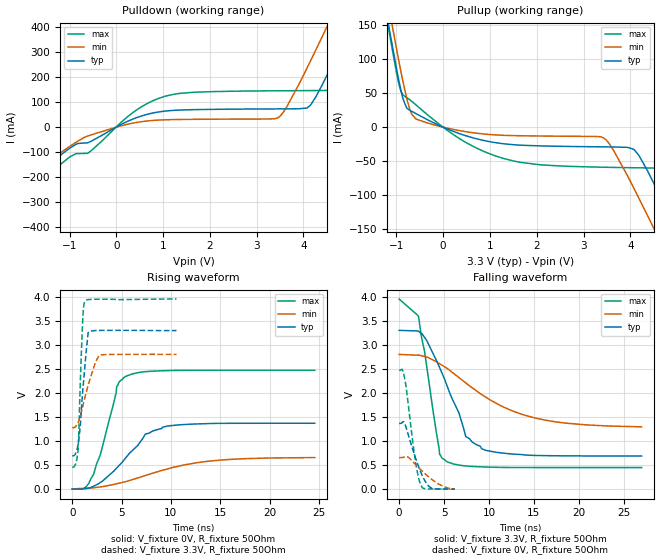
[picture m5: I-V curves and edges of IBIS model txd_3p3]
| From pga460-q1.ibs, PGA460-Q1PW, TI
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|   txd_3p3 Model
[Model]   txd_3p3
Model_type   Output
Polarity   Non-Inverting
Vmeas = 1.65
Vref = 0
Cref = 2pF
Rref = 600
|   typ   min   max
|   (nom PVT)   (fast PVT)   (slow PVT)
C_comp   1.546e-12   1.546e-12   1.546e-12
| Where nom  PVT is Nominal Process, 3.3V, 27C
|   Fast PVT is Strong Process,  3.95V, -40C
|   Slow PVT is Weak Process,   2.8V, 125C
[Voltage Range]   3.3   2.8   3.95
|Junction Temperature
[Temperature Range]   27   125   -40
[Pullup Reference]   3.3   2.8   3.95
[Pulldown Reference]   0   0   0
[Power Clamp Reference]   3.3   2.8   3.95
[GND Clamp Reference]   0   0   0
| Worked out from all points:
|   slope of the pulldown table from 0 to 0.495 V, typ, clamps not added: 11.9 ohm
|   slope of the pullup table from 0 to 0.495 V, typ, clamps not added: 38.7 ohm
|   falling waveform, V_fixture 3.3V, R_fixture 50Ohm: 20-80 % time 3.37ns typ, 7.63ns min, 1.76ns max; typ from 3.3 V to 0.689 V
|   rising waveform, V_fixture 0V, R_fixture 50Ohm: 20-80 % time 3.6ns typ, 7.01ns min, 1.99ns max; typ from 0 V to 1.37 V
|   rising waveform, V_fixture 3.3V, R_fixture 50Ohm: 20-80 % time 611ps typ, 1.23ns min, 346ps max; typ from 0.689 V to 3.29 V
|   falling waveform, V_fixture 0V, R_fixture 50Ohm: 20-80 % time 1.52ns typ, 2.39ns min, 1.01ns max; typ from 1.37 V to 0 V
[Pulldown]
|   Voltage   I(typ)   I(min)   I(max)
-3.3V     -421.7mA   -396.6mA   -469.6mA
-716.7mV  -63.75mA   -44.17mA   -104.9mA
804.8mV   57.27mA    27.04mA    107.1mA
1.647V    69.71mA    31.12mA    138.9mA
3.445V    72.68mA    36.55mA    145mA
3.633V    72.81mA    77.77mA    145.2mA
4.075V    76.37mA    235.5mA    145.7mA
4.557V    227.4mA    422.1mA    146.8mA
4.833V    334.7mA    530.8mA    152.6mA
5.046V    419.1mA    614.8mA    215mA
5.514V    608.1mA    800.5mA    399.1mA
6.6V      1.053A     1.233A     854.8mA
[Pullup]
|   Voltage   I(typ)   I(min)   I(max)
-3.3V     1.024A     1.027A     1.051A
-1.144V   141.3mA    170mA      136.2mA
-902.3mV  54.03mA    81.66mA    52.9mA
-715.6mV  24.87mA    26.75mA    40.4mA
-575.6mV  19.68mA    11.74mA    32.37mA
1.092V    -22.58mA   -11.34mA   -41.74mA
3.42V     -29.04mA   -15.47mA   -59.01mA
4.075V    -32.79mA   -89.97mA   -59.78mA
4.495V    -81.79mA   -148.1mA   -60.25mA
5.054V    -162.5mA   -227.5mA   -93.94mA
5.406V    -215mA     -277.9mA   -146.3mA
6.6V      -395.5mA   -449.7mA   -336.5mA
[Ramp]
R_load = 50
|   typ   min   max
dV/dt_r   0.820065/3.73263e-09   0.393374/7.0168e-09   1.48123/1.93337e-09
dV/dt_f   1.56675/3.49199e-09   0.910333/7.76953e-09   2.10032/1.59697e-09
[Falling Waveform]
V_fixture = 3.3V
V_fixture_min = 2.8V
V_fixture_max = 3.95V
R_fixture = 50Ohm
|   Time   V(typ)   V(min)   V(max)
0s        3.3V       2.8V       3.95V
2.119ns   3.286V     2.783V     3.603V
2.838ns   3.151V     2.757V     2.851V
4.507ns   2.524V     2.606V     720.1mV
5.295ns   2.166V     2.514V     574.8mV
6.66ns    1.58V      2.318V     501.1mV
7.409ns   1.095V     2.209V     483.2mV
9.644ns   807.1mV    1.912V     460.8mV
16.18ns   697.4mV    1.437V     449.5mV
26.98ns   688.8mV    1.296V     449.4mV
[Rising Waveform]
V_fixture = 0V
V_fixture_min = 0V
V_fixture_max = 0V
R_fixture = 50Ohm
|   Time   V(typ)   V(min)   V(max)
0s        121.9pV    1.304nV    174.6pV
1.266ns   3.223mV    13.81mV    24.73mV
2.179ns   57.89mV    24.39mV    312.4mV
2.838ns   133mV      41.85mV    707.5mV
4.507ns   435.4mV    108.2mV    2.137V
5.383ns   638.1mV    150mV      2.337V
7.409ns   1.14V      279.1mV    2.439V
9.524ns   1.303V     409.2mV    2.461V
14.98ns   1.364V     599.6mV    2.469V
24.58ns   1.367V     652.8mV    2.469V
[Rising Waveform]
V_fixture = 3.3V
V_fixture_min = 2.8V
V_fixture_max = 3.95V
R_fixture = 50Ohm
|   Time   V(typ)   V(min)   V(max)
0s        688.6mV    1.282V     449.4mV
318.6ps   725.5mV    1.293V     508.7mV
593.1ps   928.5mV    1.376V     809.6mV
836.4ps   1.36V      1.534V     2.343V
1.042ns   1.986V     1.707V     3.436V
1.125ns   2.188V     1.776V     3.752V
1.263ns   2.509V     1.89V      3.896V
1.604ns   3.25V      2.152V     3.937V
2.717ns   3.296V     2.778V     3.947V
10.57ns   3.295V     2.799V     3.95V
[Falling Waveform]
V_fixture = 0V
V_fixture_min = 0V
V_fixture_max = 0V
R_fixture = 50Ohm
|   Time   V(typ)   V(min)   V(max)
0s        1.367V     655.6mV    2.469V
338.7ps   1.387V     656.2mV    2.489V
597.3ps   1.373V     668.9mV    2.317V
818.6ps   1.253V     677.9mV    2.058V
1.763ns   681.9mV    525mV      643.9mV
2.138ns   481.9mV    453.4mV    255.5mV
2.409ns   352.5mV    403.4mV    87.82mV
3.042ns   121.4mV    293.8mV    8.441mV
3.587ns   20.96mV    210.4mV    3.346mV
6.179ns   472.8uV    4.077mV    4.167mV
